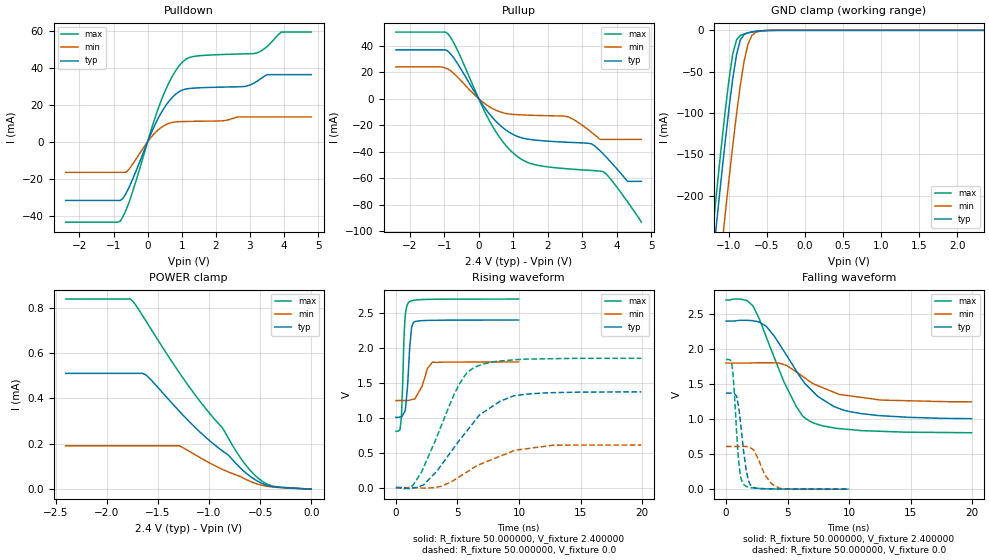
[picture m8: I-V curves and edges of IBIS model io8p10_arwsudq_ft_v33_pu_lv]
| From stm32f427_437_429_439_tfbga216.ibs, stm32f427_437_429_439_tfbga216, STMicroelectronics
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|   Model io8p10_arwsudq_ft_v33_pu_lv
[Model]  io8p10_arwsudq_ft_v33_pu_lv
Model_type I/O
Polarity   Non-Inverting
Enable   Active-Low
Vinl =   0.720000V
Vinh =   1.680000V
Vmeas =  1.200000V
Cref =   40.000000pF
Rref =   100.000000M
Vref =   0.0V
C_comp   2.828400pF   2.771400pF   2.910300pF
[Temperature Range]   25.000000   0.125000k   -40.000000
[Pullup Reference]   2.400000V   1.800000V   2.700000V
[Pulldown Reference]   0.0V   0.0V   0.0V
[POWER Clamp Reference]   2.400000V   1.800000V   2.700000V
[GND Clamp Reference]   0.0V   0.0V   0.0V
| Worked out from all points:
|   slope of the pulldown table from 0 to 0.36 V, typ, clamps not added: 25 ohm
|   slope of the pullup table from 0 to 0.36 V, typ, clamps not added: 27.7 ohm
|   GND clamp passes 1 mA (typ) near -0.62 V on its own axis
|   rising waveform, R_fixture 50.000000, V_fixture 2.400000: 20-80 % time 323ps typ, 714ps min, 222ps max; typ from 1.01 V to 2.4 V
|   rising waveform, R_fixture 50.000000, V_fixture 0.0: 20-80 % time 3.77ns typ, 4.15ns min, 2.7ns max; typ from 0.001 V to 1.37 V
|   falling waveform, R_fixture 50.000000, V_fixture 2.400000: 20-80 % time 3.65ns typ, 3.54ns min, 2.75ns max; typ from 2.4 V to 1.01 V
|   falling waveform, R_fixture 50.000000, V_fixture 0.0: 20-80 % time 553ps typ, 1.06ns min, 409ps max; typ from 1.37 V to 0.001 V
[Pulldown]
|Voltage   I(typ)   I(min)   I(max)
-2.4V     -31.66mA   -16.51mA   -43.42mA
-800mV    -31.66mA   -16.51mA   -42.86mA
-480mV    -21.98mA   -13.17mA   -29.21mA
80mV      3.63mA     1.966mA    5.014mA
480mV     18.16mA    8.738mA    26.02mA
800mV     25.38mA    10.72mA    37.77mA
1.12V     28.53mA    11.02mA    44.6mA
2.8V      29.84mA    13.46mA    47.53mA
3.2V      32.6mA     13.46mA    48.03mA
3.52V     36.33mA    13.46mA    51.75mA
3.92V     36.33mA    13.46mA    59.31mA
4.8V      36.33mA    13.46mA    59.31mA
[Pullup]
|Voltage   I(typ)   I(min)   I(max)
-2.4V     36.82mA    24mA       50.22mA
-960mV    36.82mA    23.02mA    50.22mA
-640mV    27.62mA    17.03mA    37.94mA
320mV     -11.75mA   -6.207mA   -17.08mA
640mV     -20.52mA   -10.1mA    -30.35mA
960mV     -26.47mA   -11.82mA   -40.02mA
1.52V     -30.88mA   -12.51mA   -49.05mA
2.56V     -32.88mA   -13.48mA   -52.9mA
3.28V     -34.2mA    -25.51mA   -54.17mA
3.6V      -41.33mA   -30.75mA   -54.99mA
4.32V     -62.42mA   -30.75mA   -77.88mA
4.72V     -62.42mA   -30.75mA   -93.2mA
[GND_clamp]
|Voltage   I(typ)   I(min)   I(max)
-2.4V     -1.428A    -1.51A     -1.401A
-1.2V     -266.4mA   -356.3mA   -229.4mA
-1.15V    -221.3mA   -311mA     -184.1mA
-1.1V     -177.3mA   -266.4mA   -140mA
-1.05V    -134.8mA   -222.7mA   -97.97mA
-950mV    -58.22mA   -139.2mA   -28.55mA
-900mV    -29.03mA   -100.6mA   -11.27mA
-850mV    -11.41mA   -65.77mA   -6.067mA
-750mV    -2.852mA   -16.63mA   -3.179mA
-700mV    -1.914mA   -6.318mA   -2.181mA
-600mV    -750uA     -1.167mA   -738.3uA
2.35V     0A         0A         0A
[POWER_clamp]
|Voltage   I(typ)   I(min)   I(max)
-2.4V     511uA      191.4uA    838.7uA
-1.77V    511uA      191.4uA    838.7uA
-1.74V    511uA      191.4uA    826.9uA
-1.62V    505.2uA    191.4uA    744.6uA
-1.29V    344.1uA    191.4uA    514uA
-1.08V    248.7uA    137.3uA    383.1uA
-870mV    169.3uA    87.75uA    271.7uA
-720mV    105.7uA    60.5uA     157.1uA
-570mV    47.98uA    29.54uA    70.06uA
-480mV    25.17uA    16.94uA    35.08uA
-390mV    12.49uA    10.17uA    15.15uA
0V        0A         0A         0A
[Ramp]
| variable   typ   min   max
dV/dt_r  0.82201/3.77383n   0.36585/4.15344n   1.11107/2.69969n
dV/dt_f  0.83238/3.64996n   0.33372/3.61040n   1.13579/2.75561n
R_load = 50.000000
[Rising Waveform]
R_fixture= 50.000000
V_fixture= 2.400000
V_fixture_min= 1.800000
V_fixture_max= 2.700000
|time   V(typ)   V(min)   V(max)
0s        1.007V     1.247V     806mV
320.3ps   1.012V     1.247V     824.6mV
440.4ps   1.017V     1.247V     998.1mV
720.7ps   1.092V     1.247V     2.372V
940.9ps   1.446V     1.247V     2.624V
1.041ns   1.757V     1.25V      2.652V
1.281ns   2.3V       1.26V      2.675V
1.441ns   2.368V     1.267V     2.682V
2.963ns   2.396V     1.795V     2.696V
9.97ns    2.4V       1.8V       2.7V
[Rising Waveform]
R_fixture= 50.000000
V_fixture= 0.0
V_fixture_min= 0.0
V_fixture_max= 0.0
|time   V(typ)   V(min)   V(max)
0s        956.5uV    874.7uV    1.143mV
1.361ns   -5.414mV   361.4uV    30.76mV
2.082ns   28.52mV    -5.67mV    222.5mV
4.765ns   583.3mV    112.7mV    1.349V
5.566ns   767.5mV    202.2mV    1.597V
6.326ns   937.1mV    287.2mV    1.715V
8.448ns   1.235V     448.8mV    1.814V
9.57ns    1.314V     528.3mV    1.829V
12.77ns   1.36V      607.7mV    1.846V
19.94ns   1.371V     610.3mV    1.852V
[Falling Waveform]
R_fixture= 50.000000
V_fixture= 2.400000
V_fixture_min= 1.800000
V_fixture_max= 2.700000
|time   V(typ)   V(min)   V(max)
0s        2.4V       1.8V       2.7V
1.682ns   2.41V      1.8V       2.693V
2.202ns   2.403V     1.802V     2.61V
3.283ns   2.322V     1.805V     2.165V
4.725ns   1.964V     1.776V     1.525V
6.166ns   1.568V     1.618V     1.058V
6.847ns   1.43V      1.532V     966.9mV
8.729ns   1.184V     1.386V     876.4mV
10.13ns   1.105V     1.331V     849.9mV
19.94ns   1.007V     1.247V     806mV
[Falling Waveform]
R_fixture= 50.000000
V_fixture= 0.0
V_fixture_min= 0.0
V_fixture_max= 0.0
|time   V(typ)   V(min)   V(max)
0s        1.371V     610.3mV    1.852V
460.5ps   1.371V     610.2mV    1.791V
660.7ps   1.367V     610.1mV    1.413V
1.041ns   1.153V     609.9mV    371.2mV
1.481ns   470.1mV    610.9mV    61.26mV
1.822ns   123mV      606.8mV    29.71mV
2.302ns   21.77mV    542.6mV    16.15mV
3.143ns   6.954mV    207.9mV    7.339mV
4.364ns   3.523mV    11.87mV    3.113mV
9.97ns    956.5uV    874.7uV    1.143mV
